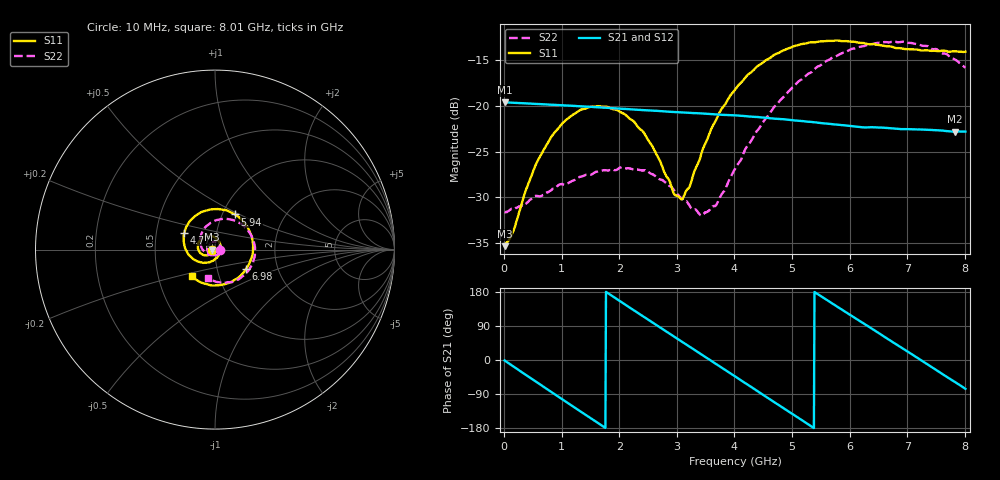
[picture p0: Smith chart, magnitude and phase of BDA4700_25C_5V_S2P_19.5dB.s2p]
!Agilent Technologies,E5071B,MY42404982,A.09.10
!Date: Mon Oct 20 13:36:07 2025
!Data & Calibration Information:
!Freq	S11:SOLT2(ON)	S21:SOLT2(ON)	S12:SOLT2(ON)	S22:SOLT2(ON)
# Hz S RI R 50
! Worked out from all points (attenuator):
!   801 points, 10 MHz to 8.01 GHz, reference 50 ohm
!   highest |S21| = -19.59 dB at 10 MHz (marker M1); lowest = -22.8 dB at 7.83 GHz (marker M2)
!   lowest |S11| = -35.3 dB at 10 MHz (marker M3), VSWR 1.03, Z = 48.3 - j0.107 ohm
!   |S11| at or under -10 dB: start of sweep to end of sweep
!   |S22| runs from -32.0 to -13.0 dB; largest |S21 - S12| = 0.00084
!   S11 on the Smith chart (normalised r, x): 10 MHz: 0.97, -0.00; 4.77 GHz: 0.70, +0.14; 5.94 GHz: 1.15, +0.47; 6.98 GHz: 1.38, -0.31; 8.01 GHz: 0.74, -0.23
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1e7  -0.0171 -0.00111  0.1048 -0.00227  0.1048 -0.00238  0.0262 -0.000863
1.5e8  -0.0181 -0.00918  0.1001 -0.0283  0.1 -0.0283  0.0263 -0.00723
4.3e8  -0.0283 -0.0255  0.0734 -0.0722  0.0734 -0.0722  0.0195 -0.0229
7e8  -0.0483 -0.0326  0.0314 -0.097  0.0314 -0.097  0.00548 -0.0326
1.02e9  -0.0773 -0.0231  -0.0253 -0.0975  -0.0254 -0.0976  -0.0169 -0.0332
1.35e9  -0.0955 0.00633  -0.0738 -0.0666  -0.0738 -0.0666  -0.0374 -0.0169
2.09e9  -0.0492 0.0757  -0.0812 0.0516  -0.0813 0.0516  -0.0277 0.0364
2.42e9  -0.00609 0.0716  -0.0395 0.0861  -0.0395 0.0861  -0.00182 0.0443
2.68e9  0.0207 0.0477  0.00194 0.0938  0.00198 0.0938  0.0162 0.0365
2.95e9  0.0314 0.0104  0.0435 0.0817  0.0435 0.0816  0.0277 0.0207
3.1e9  0.0285 -0.0122  0.0627 0.0673  0.0626 0.0675  0.0298 0.0082
3.46e9  -0.00551 -0.0587  0.089 0.0179  0.089 0.0179  0.0168 -0.0193
3.69e9  -0.0443 -0.0724  0.088 -0.0177  0.088 -0.0179  -0.00177 -0.0288
4.01e9  -0.1059 -0.0613  0.0647 -0.0607  0.0647 -0.0607  -0.0358 -0.0274
4.77e9  -0.1704 0.0942  -0.0411 -0.0742  -0.0408 -0.0744  -0.0818 0.0658
5.35e9  -0.066 0.2124  -0.0814 -0.00486  -0.0814 -0.00515  -0.0138 0.1533
5.94e9  0.1122 0.1961  -0.0453 0.0636  -0.0455 0.0635  0.1233 0.1543
6.68e9  0.2109 -0.0144  0.0445 0.061  0.0448 0.0609  0.2225 -0.00771
6.98e9  0.1739 -0.1072  0.0676 0.0315  0.0677 0.0312  0.2036 -0.088
7.43e9  0.0513 -0.193  0.0698 -0.0242  0.0697 -0.0245  0.1118 -0.1716
7.83e9  -0.08 -0.1821  0.0381 -0.0614  0.0381 -0.0615  0.00457 -0.1793
8.01e9  -0.1296 -0.1496  0.0174 -0.0702  0.0174 -0.0702  -0.038 -0.157
